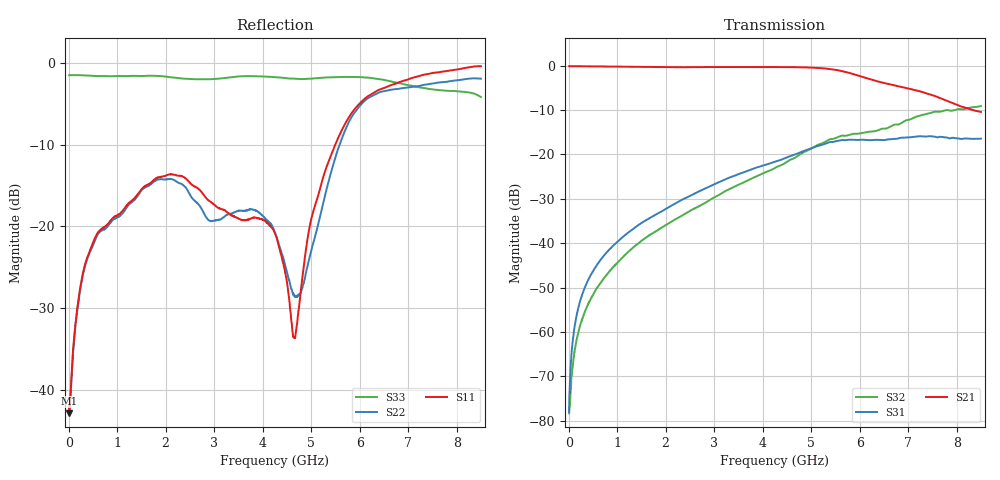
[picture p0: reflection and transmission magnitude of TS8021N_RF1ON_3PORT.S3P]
!Agilent Technologies,E5071C,MY46522130,B.12.04
!Date: Mon Jun 30 18:14:17 2025
!Data & Calibration Information:
!Freq	S11:SOLT4(ON)	S12:SOLT4(ON)	S13:SOLT4(ON)
!	S21:SOLT4(ON)	S22:SOLT4(ON)	S23:SOLT4(ON)
!	S31:SOLT4(ON)	S32:SOLT4(ON)	S33:SOLT4(ON)
!PortZ  Port1:50+j0  Port2:50+j0  Port3:50+j0
!Above PortZ is port z conversion or system Z0 setting when saving the data.
!When reading, reference impedance value at option line is always used.
# Hz S dB R 50
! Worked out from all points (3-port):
!   1601 points, 10 MHz to 8.5 GHz, reference 50 ohm
!   strongest paths, dB at 10 MHz, 2.132 GHz, 4.255 GHz, 6.378 GHz, 8.5 GHz:
!     S21: -0.1, -0.4, -0.3, -3.6, -10.4
!     S31: -78.0, -31.5, -21.6, -16.7, -16.4
!     S32: -78.4, -35.1, -23.1, -14.6, -9.1
!   lowest |S11| = -42.9 dB at 15.31 MHz (marker M1), VSWR 1.01, Z = 50.7 - j0.208 ohm
!   |S11| at or under -10 dB: start of sweep to 5.498 GHz
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1e7  -42.11 -5.4  -0.12 -0.2  -77.23 46.7
     -0.12 -0.2  -42.10 -5.1  -80.45 31.3
     -78.02 45.9  -78.36 31.6  -1.50 179.8
1.530625e7  -42.90 -16.7  -0.12 -0.3  -75.89 60.2
            -0.12 -0.3  -42.48 -17.0  -79.00 36.2
            -74.58 59.8  -77.13 37.8  -1.50 179.7
2.169438e8  -28.37 -83.4  -0.13 -4.3  -53.85 89.2
            -0.12 -4.3  -28.69 -87.2  -59.33 89.3
            -53.92 89.2  -59.44 89.7  -1.51 177.9
7.95325e8  -19.79 -97.9  -0.19 -15.6  -41.95 93.1
           -0.19 -15.6  -20.05 -107.6  -46.92 101.7
           -41.96 93.0  -46.97 101.4  -1.62 168.2
2.1325e9  -13.65 -108.6  -0.35 -40.8  -31.45 90.8
          -0.35 -40.9  -14.24 -146.2  -35.04 101.3
          -31.48 90.6  -35.08 101.1  -1.77 146.8
4.255e9  -20.88 -138.6  -0.32 -86.1  -21.59 62.1
         -0.31 -86.2  -20.77 156.9  -22.96 80.3
         -21.65 62.1  -23.07 81.1  -1.76 105.0
4.658275e9  -33.67 145.0  -0.34 -96.6  -19.96 54.8
            -0.34 -96.7  -28.58 -165.0  -20.59 75.5
            -20.06 54.6  -20.80 75.3  -1.93 99.7
5.024406e9  -18.63 77.0  -0.45 -107.4  -18.54 45.4
            -0.45 -107.4  -22.43 -134.1  -18.41 66.9
            -18.57 45.2  -18.54 66.5  -1.91 91.7
5.830956e9  -6.18 88.2  -1.77 -134.9  -16.80 17.9
            -1.78 -135.0  -6.66 170.1  -15.60 37.4
            -16.69 17.9  -15.46 37.0  -1.72 85.1
8.5e9  -0.41 59.8  -10.47 -174.1  -16.49 -30.5
       -10.44 -174.4  -1.93 112.0  -9.33 -30.5
       -16.44 -30.3  -9.10 -30.4  -4.18 52.9
